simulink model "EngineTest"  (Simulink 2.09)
settings: Solver=ode45  StartTime=0.0  StopTime=999999  MaxStep=10  RelTol=1e-3  AbsTol=1e-3
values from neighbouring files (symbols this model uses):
  Fe0 = Fi+gamma*sqrt(theta0)    [VdataM.m]
  Fi = 1000    [VdataM.m]
  gamma = 12500    [VdataM.m]
  gamma1 = 0    [VdataM.m]
  gamma3 = 0    [VdataM.m]
  T = 2.5    [HdataF.m]    (also in Mdata.m = 0.5; Mdata25.m = 0.5; VdataC.m = 0.25; VdataF.m = 0.25)
  te_n = 0.1    [VdataM.m]
  te_p = 1    [VdataM.m]

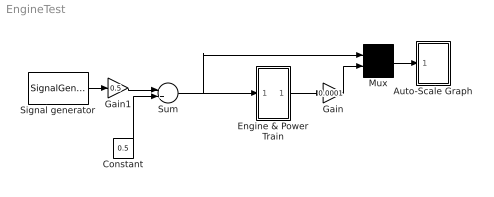
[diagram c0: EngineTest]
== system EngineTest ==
  Auto-Scale Graph : Subsystem  mask(Storage scope.){}
      mask help: Storage scope using MATLAB graph window. Enter plotting ranges and line type.
      mask init:
      | npts = @4; color = @5; ax = [0, @1, @2, @3]; dt=@6;
  Constant : Constant  Value=0.5
  Engine & Power Train : Subsystem
  Gain : Gain  Gain=0.0001
  Gain1 : Gain  Gain=0.5
  Mux : Mux  Inputs=2
  Signal generator : SignalGenerator  WaveForm=square  Amplitude=1.000000  Frequency=1.000000  Units=rad/sec
  Sum : Sum  Inputs=++
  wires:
  Gain1/1 -> Sum/1
  Signal generator/1 -> Gain1/1
  Constant/1 -> Sum/2
  Gain/1 -> Mux/2
  Engine & Power Train/1(Engine Force_) -> Gain/1
  Mux/1 -> Auto-Scale Graph/1(x)
  Sum/1 -> Mux/1, Engine & Power Train/1(theta)

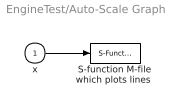
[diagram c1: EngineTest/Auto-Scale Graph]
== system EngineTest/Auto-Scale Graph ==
  x : Inport  Port=1  PortWidth=-1  SampleTime=-1
  "S-function M-file which plots lines " : S-Function  FunctionName=sfunyst  Parameters=ax, color, npts, dt
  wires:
  x/1 -> "S-function M-file which plots lines "/1

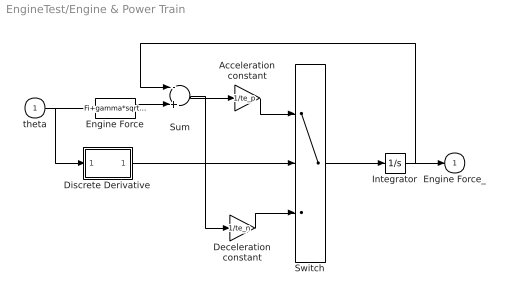
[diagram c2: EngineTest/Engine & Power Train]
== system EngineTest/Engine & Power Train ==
  theta : Inport  Port=1  PortWidth=-1  SampleTime=-1
  Acceleration constant : Gain  Gain=1/te_p
  Deceleration constant : Gain  Gain=1/te_n
  Discrete Derivative : Subsystem
  Engine Force : Fcn  Expr=Fi+gamma*sqrt(u[1])-gamma1*u[1]-gamma3*u[1]*u[1]*u[1]
  Integrator : Integrator  ExternalReset=none  InitialConditionSource=internal  InitialCondition=Fe0  LimitOutput=off  UpperSaturationLimit=inf  LowerSaturationLimit=-inf  ShowSaturationPort=off  ShowStatePort=off  AbsoluteTolerance=auto
  Sum : Sum  Inputs=-+
  Switch : Switch  Threshold=0
  Engine Force_ : Outport  Port=1  InitialOutput=0
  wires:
  theta/1 -> Discrete Derivative/1(e), Engine Force/1
  Discrete Derivative/1(ce) -> Switch/2
  Sum/1 -> Acceleration constant/1, Deceleration constant/1
  Acceleration constant/1 -> Switch/1
  Deceleration constant/1 -> Switch/3
  Switch/1 -> Integrator/1
  Integrator/1 -> Engine Force_/1, Sum/1
  Engine Force/1 -> Sum/2

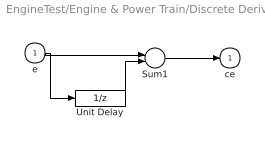
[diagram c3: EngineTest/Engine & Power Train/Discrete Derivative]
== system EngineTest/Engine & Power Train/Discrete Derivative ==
  e : Inport  Port=1  PortWidth=-1  SampleTime=-1
  Sum1 : Sum  Inputs=+-
  Unit Delay : UnitDelay  X0=0  SampleTime=T
  ce : Outport  Port=1  InitialOutput=0
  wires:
  e/1 -> Unit Delay/1, Sum1/1
  Sum1/1 -> ce/1
  Unit Delay/1 -> Sum1/2
